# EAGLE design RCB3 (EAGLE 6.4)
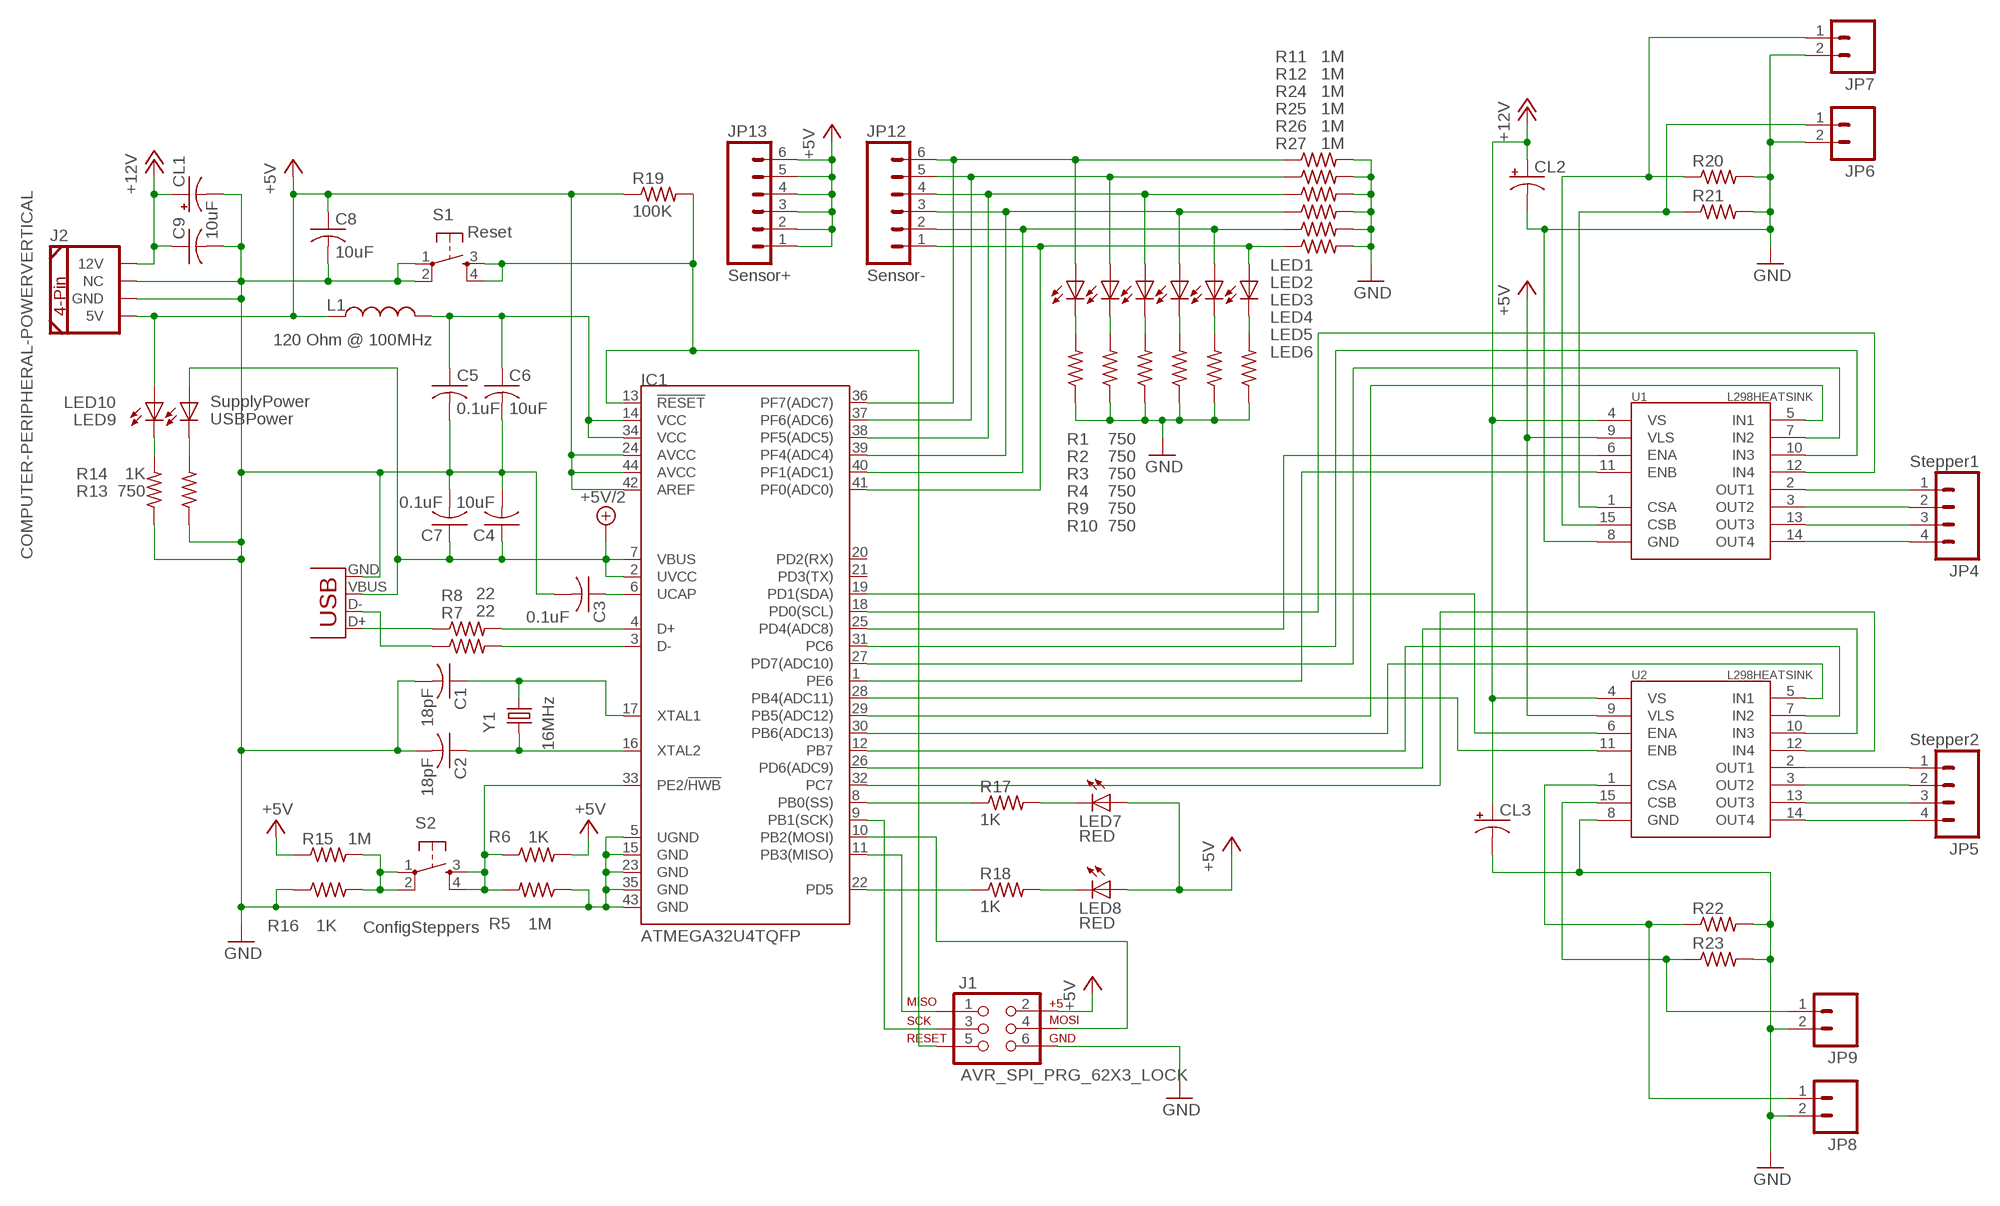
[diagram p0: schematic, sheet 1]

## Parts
C1  18pF  C-USC0603  [C0603]
C2  18pF  C-USC0603  [C0603]
C3  0.1uF  C-USC0603  [C0603]
C4  10uF  C-USC0805  [C0805]
C5  0.1uF  C-USC0603  [C0603]
C6  10uF  C-USC0805  [C0805]
C7  0.1uF  C-USC0603  [C0603]
C8  10uF  C-USC0805  [C0805]
C9  10uF  C-USC0805  [C0805]
CL1  CAP_G  [PANASONIC_G]
CL2  CAP_G  [PANASONIC_G]
CL3  CAP_G  [PANASONIC_G]
IC1  ATMEGA32U4TQFP  [SPARKFUN-DIGITALIC_TQFP44]
J1  AVR_SPI_PRG_62X3_LOCK  [2X3_LOCK]
J2  COMPUTER-PERIPHERAL-POWERVERTICAL  [COMPUTER-PERIPHERAL-POWER]
JP1  USBPTH-VERTICAL  [USB-B-PTH-VERTICAL]
JP4  Stepper1  M04POLAR  [MOLEX-1X4]
JP5  Stepper2  M04POLAR  [MOLEX-1X4]
JP6  M02LOCK  [1X02_LOCK]
JP7  M02LOCK  [1X02_LOCK]
JP8  M02LOCK  [1X02_LOCK]
JP9  M02LOCK  [1X02_LOCK]
JP12  Sensor-  M06LOCK  [1X06_LOCK]
JP13  Sensor+  M06LOCK  [1X06_LOCK]
L1  120 Ohm @ 100MHz  INDUCTOR0603  [0603]
LED1  GREEN  LED-GREEN0603  [LED-0603]
LED2  GREEN  LED-GREEN0603  [LED-0603]
LED3  GREEN  LED-GREEN0603  [LED-0603]
LED4  GREEN  LED-GREEN0603  [LED-0603]
LED5  GREEN  LED-GREEN0603  [LED-0603]
LED6  GREEN  LED-GREEN0603  [LED-0603]
LED7  RED  LED0603  [LED-0603]
LED8  RED  LED0603  [LED-0603]
LED9  USBPower  LED0603  [LED-0603]
LED10  SupplyPower  LED0603  [LED-0603]
R1  750  R-US_R0603  [R0603]
R2  750  R-US_R0603  [R0603]
R3  750  R-US_R0603  [R0603]
R4  750  R-US_R0603  [R0603]
R5  1M  R-US_R0603  [R0603]
R6  1K  R-US_R0603  [R0603]
R7  22  R-US_R0603  [R0603]
R8  22  R-US_R0603  [R0603]
R9  750  R-US_R0603  [R0603]
R10  750  R-US_R0603  [R0603]
R11  1M  R-US_R0603  [R0603]
R12  1M  R-US_R0603  [R0603]
R13  750  R-US_R0603  [R0603]
R14  1K  R-US_R0603  [R0603]
R15  1M  R-US_R0603  [R0603]
R16  1K  R-US_R0603  [R0603]
R17  1K  R-US_R0603  [R0603]
R18  1K  R-US_R0603  [R0603]
R19  100K  R-US_R0603  [R0603]
R20  R-US_R0603  [R0603]
R21  R-US_R0603  [R0603]
R22  R-US_R0603  [R0603]
R23  R-US_R0603  [R0603]
R24  1M  R-US_R0603  [R0603]
R25  1M  R-US_R0603  [R0603]
R26  1M  R-US_R0603  [R0603]
R27  1M  R-US_R0603  [R0603]
S1  Reset  TAC_SWITCHSMD  [TACTILE_SWITCH_SMD]
S2  ConfigSteppers  TAC_SWITCHSMD  [TACTILE_SWITCH_SMD]
U1  L298HEATSINK  [MULTIWATT15_6400BGHEATSINK]
U2  L298HEATSINK  [MULTIWATT15_6400BGHEATSINK]
Y1  16MHz  CRYSTALHC49UV  [HC49U-V]

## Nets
+5V: C8.1 IC1.24(AVCC) IC1.42(AREF) IC1.44(AVCC) J1.2 J2.5V JP13.1 JP13.2 JP13.3 JP13.4 JP13.5 JP13.6 L1.1 LED7.A LED8.A LED10.A R6.2 R15.1 R19.1 U1.9(VLS) U2.9(VLS)
+5V/2: C4.1 C7.1 IC1.2(UVCC) IC1.7(VBUS) JP1.VBUS LED9.A
+12V: C9.1 CL1.+(CAP+) CL2.+(CAP+) CL3.+(CAP+) J2.12V U1.4(VS) U2.4(VS)
GND: C1.2 C2.2 C3.2 C4.2 C5.2 C6.2 C7.2 C8.2 C9.2 CL1.-(CAP-) CL2.-(CAP-) CL3.-(CAP-) IC1.5(UGND) IC1.15(GND) IC1.23(GND) IC1.35(GND) IC1.43(GND) J1.6 J2.GND J2.NC JP1.GND JP6.2 JP7.2 JP8.2 JP9.2 R1.1 R2.1 R3.1 R4.1 R5.1 R9.1 R10.1 R11.2 R12.2 R13.1 R14.1 R16.1 R20.2 R21.2 R22.2 R23.2 R24.2 R25.2 R26.2 R27.2 S1.1 S1.2 U1.8(GND) U2.8(GND)
N$1: IC1.11(PB3(MISO)) J1.1
N$2: IC1.9(PB1(SCK)) J1.3
N$3: IC1.10(PB2(MOSI)) J1.4
N$4: IC1.13(!RESET) J1.5 R19.2 S1.3 S1.4
N$5: IC1.41(PF0(ADC0)) JP12.1 LED6.A R27.1
N$6: IC1.40(PF1(ADC1)) JP12.2 LED5.A R26.1
N$7: IC1.39(PF4(ADC4)) JP12.3 LED4.A R25.1
N$8: IC1.38(PF5(ADC5)) JP12.4 LED3.A R24.1
N$9: JP1.D+ R8.1
N$10: IC1.4(D+) R8.2
N$11: IC1.3(D-) R7.2
N$12: JP1.D- R7.1
N$13: C2.1 IC1.16(XTAL2) Y1.1
N$14: C1.1 IC1.17(XTAL1) Y1.2
N$15: IC1.33(PE2/!HWB) R5.2 R6.1 S2.3 S2.4
N$16: C3.1 IC1.6(UCAP)
N$17: R15.2 R16.2 S2.1 S2.2
N$18: LED8.C R18.2
N$19: LED7.C R17.2
N$20: LED1.C R1.2
N$21: LED2.C R2.2
N$22: C5.1 C6.1 IC1.14(VCC) IC1.34(VCC) L1.2
N$23: LED9.C R13.2
N$24: LED10.C R14.2
N$25: JP5.1 U2.2(OUT1)
N$26: JP5.3 U2.13(OUT3)
N$27: JP5.2 U2.3(OUT2)
N$28: JP5.4 U2.14(OUT4)
N$29: JP4.4 U1.14(OUT4)
N$30: JP4.3 U1.13(OUT3)
N$31: JP4.2 U1.3(OUT2)
N$32: JP4.1 U1.2(OUT1)
N$33: IC1.22(PD5) R18.1
N$34: IC1.8(PB0(SS)) R17.1
N$37: JP8.1 R22.1 U2.1(CSA)
N$38: JP9.1 R23.1 U2.15(CSB)
N$39: JP6.1 R21.1 U1.1(CSA)
N$40: JP7.1 R20.1 U1.15(CSB)
N$41: IC1.29(PB5(ADC12)) U1.5(IN1)
N$42: IC1.27(PD7(ADC10)) U1.7(IN2)
N$43: IC1.31(PC6) U1.10(IN3)
N$44: IC1.18(PD0(SCL)) U1.12(IN4)
N$45: IC1.30(PB6(ADC13)) U2.5(IN1)
N$46: IC1.12(PB7) U2.7(IN2)
N$47: IC1.26(PD6(ADC9)) U2.10(IN3)
N$48: IC1.32(PC7) U2.12(IN4)
N$49: IC1.36(PF7(ADC7)) JP12.6 LED1.A R11.1
N$50: IC1.37(PF6(ADC6)) JP12.5 LED2.A R12.1
N$51: IC1.25(PD4(ADC8)) U1.6(ENA)
N$52: IC1.1(PE6) U1.11(ENB)
N$53: IC1.19(PD1(SDA)) U2.6(ENA)
N$54: IC1.28(PB4(ADC11)) U2.11(ENB)
N$55: LED3.C R3.2
N$56: LED4.C R4.2
N$57: LED5.C R9.2
N$58: LED6.C R10.2
Unconnected: IC1.20(PD2(RX)) IC1.21(PD3(TX))

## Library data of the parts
C1-C4 C6 C8 = resistor:C-US: CAPACITOR, American symbol
C5 C7 C9 = rcl:C-US: CAPACITOR, American symbol
CL1-CL3 = PanasonicSMDCapLib:CAP_G: Panasonic Aluminum Electrolytic Capacitors/ HA
IC1 = SparkFun-DigitalIC:ATMEGA32U4: Atmel 44-pin 8-bit Microcontroller with 32KBytes of ISP Flash and USB Controller
J1 = SparkFun-Connectors:AVR_SPI_PRG_6: AVR ISP 6 Pin This is the reduced ISP connector for AVR programming. Common on Arduino. This footprint will take up less PCB space and can be used with a 10-pin to 6-pin adapter such as SKU: BOB-08508
J2 = SparkFun-Connectors:COMPUTER-PERIPHERAL-POWER
JP1 = SparkFun-Connectors:USB: USB Connectors USB-B-PTH is fully proven SKU : PRT-00139/CONN-08278 USB-miniB is fully proven SKU : PRT-00587 USB-A-PCB is untested. USB-A-H is throughly reviewed, but untested. Spark Fun Electronics SKU : PRT-00437 USB-B-SMT is throughly reviewed, but untested. Needs silkscreen touching up.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
JP4 JP5 = SparkFun-Connectors:M04: Header 4 Standard 4-pin 0.1" header. Use with straight break away headers (SKU : PRT-00116), right angle break away headers (PRT-00553), swiss pins (PRT-00743), machine pins (PRT-00117), and female headers (PRT-00115). Molex polarized connector foot print use with SKU : PRT-08231 with associated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
JP6-JP9 = SparkFun-Connectors:M02: Header 2
JP12 JP13 = SparkFun-Connectors:M06: Header 6 Standard 6-pin 0.1" header. Use with straight break away headers (SKU : PRT-00116), right angle break away headers (PRT-00553), swiss pins (PRT-00743), machine pins (PRT-00117), and female headers (PRT-00115). Molex polarized connector foot print use with SKU : PRT-08094 with associated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
L1 = SparkFun-Passives:INDUCTOR: Inductors
LED1-LED6 = SparkFun-LED:LED-GREEN: Various green LEDs; PROD_ID: DIO-00821
LED7-LED10 = SparkFun:LED: LEDs
R1-R6 R9-R12 R24-R27 = resistor:R-US_: RESISTOR, American symbol
R7 R8 R13-R23 = rcl:R-US_: RESISTOR, American symbol
S1 S2 = SparkFun:TAC_SWITCH: Momentary Switch Button commonly used for reset or general input. Spark Fun Electronics SKU : COM-00097
U1 U2 = SparkFun-PowerIC:L298: L298 Dual Full Bridge Driver
Y1 = SparkFun:CRYSTAL: Crystals

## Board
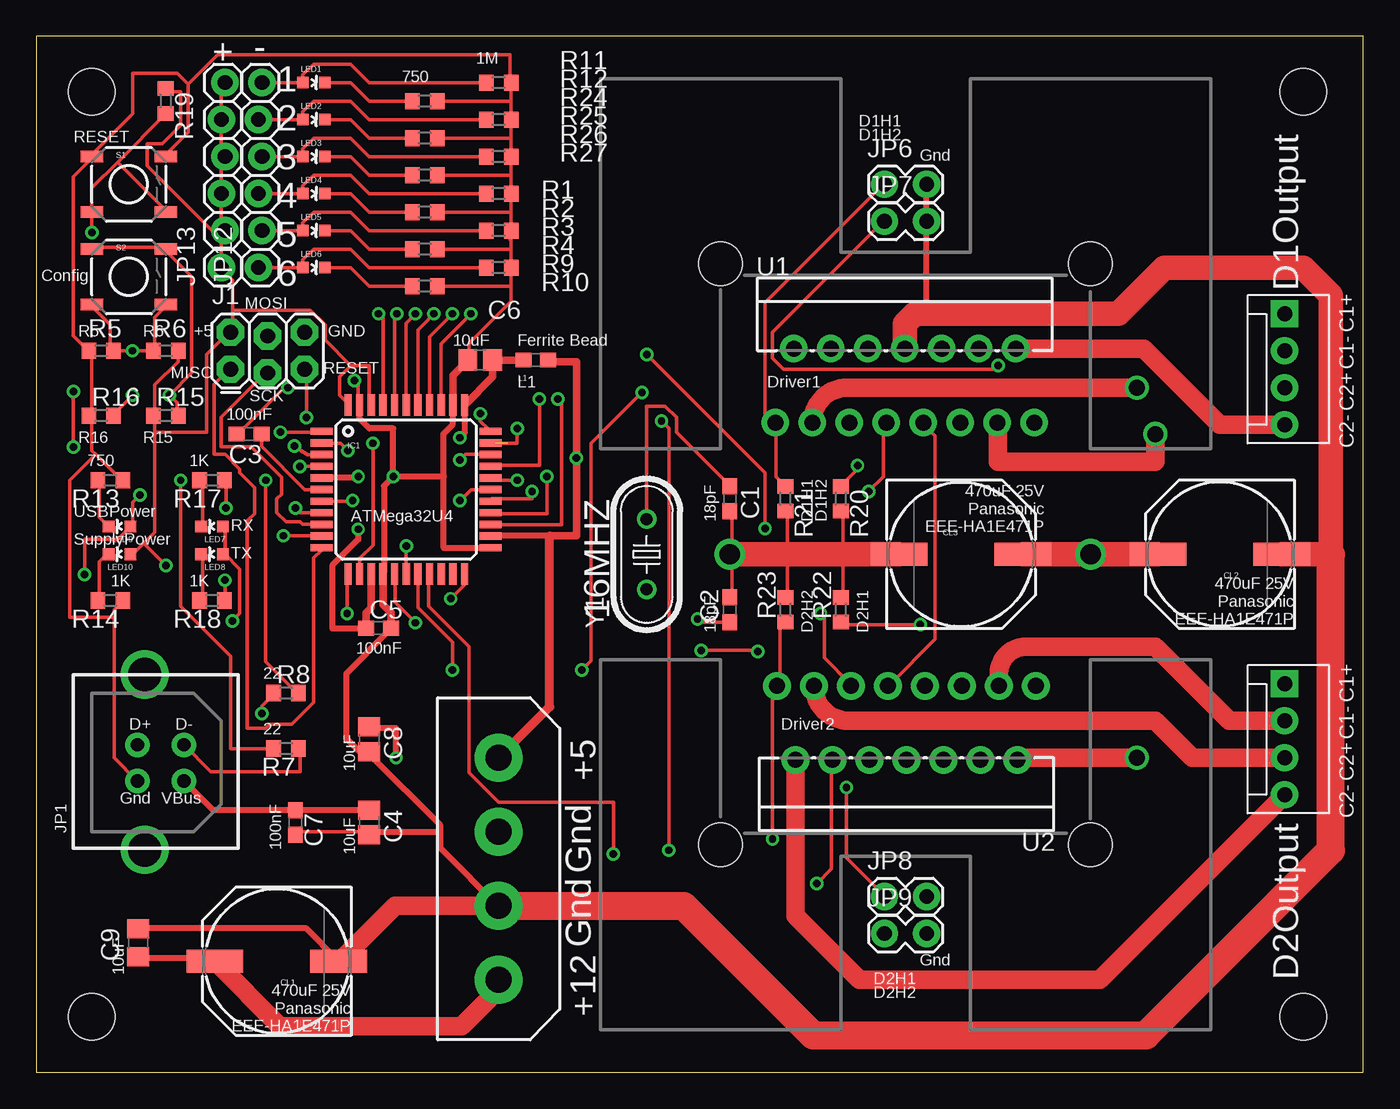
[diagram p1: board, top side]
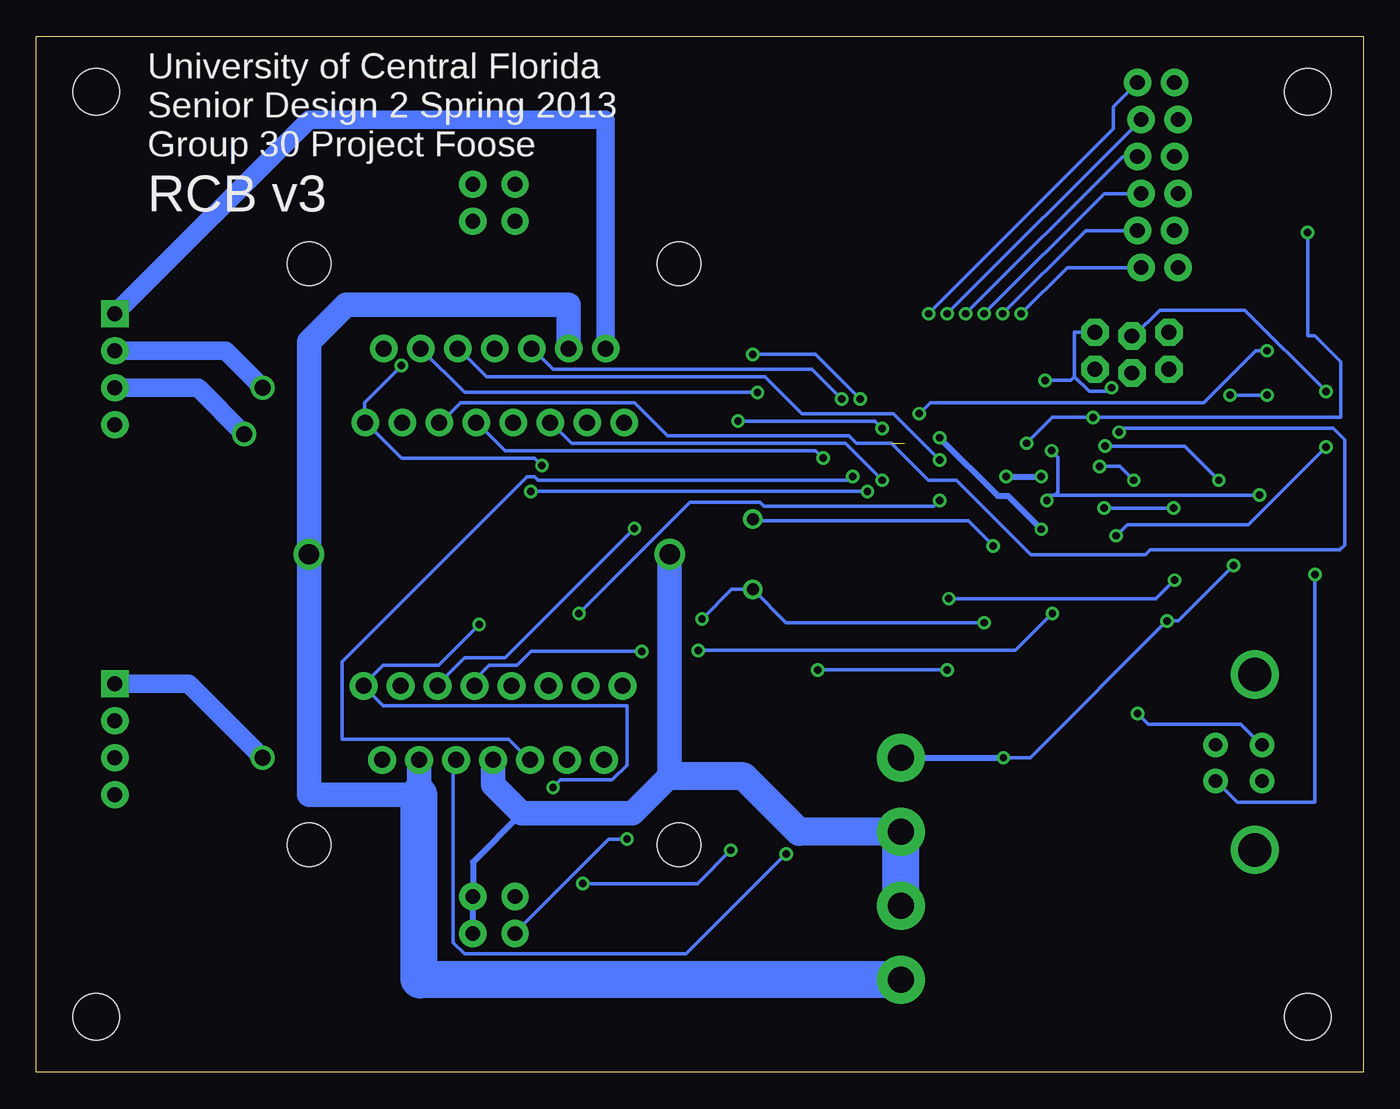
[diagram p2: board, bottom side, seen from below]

Size 91.11 x 71.11 mm. Coordinates in mm from the lower left corner, seen from the top.
Outline: 0,0 91.11,0 91.11,71.11 0,71.11 0,0
Copper layers (1*16): Top 0.035mm / dielectric 1.5mm / Bottom 0.035mm
Design rules "default *": minimum track width 10mil, minimum drill 20mil, track to track 8mil, track to pad 10mil, pad to pad 10mil, via to via 10mil, smd to smd 8mil, copper to edge 40mil, drill to drill 8mil, minimum pad ring 10mil, minimum via ring 8mil, stop-mask expansion 4mil, vias tented up to drill 0mil, thermal gap 10mil
Holes 3.2 mm at 3.81,3.81 3.81,67.31 87,67.31 87,3.81

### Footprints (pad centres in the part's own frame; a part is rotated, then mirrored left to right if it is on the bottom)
C0603 = smd 1.1 x 1: 1 -0.85,0; 2 0.85,0
C0805 = smd 1.3 x 1.5: 1 -0.85,0; 2 0.85,0
C0805' = smd 1.3 x 1.5: 1 -0.95,0; 2 0.95,0
PANASONIC_G = smd 3.9 x 1.6: + 4.25,0; - -4.25,0
SPARKFUN-DIGITALIC_TQFP44 = smd 1.5 x 0.5: 1 -5.8,4; 2 -5.8,3.2; 3 -5.8,2.4; 4 -5.8,1.6; 5 -5.8,0.8; 6 -5.8,0; 7 -5.8,-0.8; 8 -5.8,-1.6; 9 -5.8,-2.4; 10 -5.8,-3.2; 11 -5.8,-4; 23 5.8,-4; 24 5.8,-3.2; 25 5.8,-2.4; 26 5.8,-1.6; 27 5.8,-0.8; 28 5.8,0; 29 5.8,0.8; 30 5.8,1.6; 31 5.8,2.4; 32 5.8,3.2; 33 5.8,4 | smd 0.5 x 1.5: 12 -4,-5.8; 13 -3.2,-5.8; 14 -2.4,-5.8; 15 -1.6,-5.8; 16 -0.8,-5.8; 17 0,-5.8; 18 0.8,-5.8; 19 1.6,-5.8; 20 2.4,-5.8; 21 3.2,-5.8; 22 4,-5.8; 34 4,5.8; 35 3.2,5.8; 36 2.4,5.8; 37 1.6,5.8; 38 0.8,5.8; 39 0,5.8; 40 -0.8,5.8; 41 -1.6,5.8; 42 -2.4,5.8; 43 -3.2,5.8; 44 -4,5.8
2X3_LOCK = drill 1.016 pad 1.88 octagon: 1 0,0; 2 0,2.54; 3 2.54,-0.254; 4 2.54,2.286; 5 5.08,0; 6 5.08,2.54
COMPUTER-PERIPHERAL-POWER = drill 1.778 pad 3.302: 5V 7.62,0; 12V -7.62,0; GND 2.54,0; NC -2.54,0
USB-B-PTH-VERTICAL = drill 0.914 pad 1.676: D+ 4.826,4.394; D- 4.826,7.595; GND 7.315,4.394; VBUS 7.315,7.595 | drill 2.286: P$1 0,4.902; P$2 12.04,4.902
MOLEX-1X4 = drill 1.016 pad 1.88 square: 1 0,0 | drill 1.016 pad 1.88: 2 2.54,0; 3 5.08,0; 4 7.62,0
1X02_LOCK = drill 1.016 pad 1.88: 1 -0.178,0; 2 2.718,0
1X06_LOCK = drill 1.016 pad 1.88: 1 0,0; 2 2.54,-0.254; 3 5.08,0; 4 7.62,-0.254; 5 10.16,0; 6 12.7,-0.254
0603 = smd 1.1 x 1: 1 -0.85,0; 2 0.85,0
LED-0603 = smd 0.8 x 0.8: A 0,-0.75; C 0,0.75
R0603 = smd 1 x 1.1: 1 -0.85,0; 2 0.85,0
TACTILE_SWITCH_SMD = smd 1.524 x 0.762: 1 -2.54,1.905; 2 2.54,1.905; 3 -2.54,-1.905; 4 2.54,-1.905
MULTIWATT15_6400BGHEATSINK = drill 1.1 pad 1.9: 1 -8.95,-2.39; 2 -7.68,2.69; 3 -6.41,-2.39; 4 -5.14,2.69; 5 -3.87,-2.39; 6 -2.6,2.69; 7 -1.33,-2.39; 8 -0.06,2.69; 9 1.21,-2.39; 10 2.48,2.69; 11 3.75,-2.39; 12 5.02,2.69; 13 6.29,-2.39; 14 7.56,2.69; 15 8.83,-2.39 | hole 2.997: -12.7,8.509; 12.7,8.509
HC49U-V = drill 0.813: 1 -2.413,0; 2 2.413,0

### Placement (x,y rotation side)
C1  47.62,39.37 270 top
C2  47.62,31.75 90 top
C3  14.61,43.81 180 top
C4  22.86,17.14 270 top
C5  23.5,30.48 0 top
C6  30.48,48.9 180 top
C7  17.78,17.14 270 top
C8  22.86,22.86 270 top
C9  10uF  [C0805']  6.99,8.89 90 top
CL1  16.51,7.62 180 top
CL2  81.28,35.56 180 top
CL3  63.5,35.56 0 top
IC1  25.4,40.01 0 top
J1  13.34,48.26 0 top
J2  31.75,13.97 90 top
JP1  2.54,27.3 270 top
JP4  85.72,52.07 270 top
JP5  85.72,26.67 270 top
JP6  58.42,60.96 0 top
JP7  58.42,58.42 0 top
JP8  58.42,12.06 0 top
JP9  58.42,9.53 0 top
JP12  15.24,55.24 90 top
JP13  12.7,55.24 90 top
L1  34.29,48.9 180 top
LED1  19.05,67.94 270 top
LED2  19.05,65.41 270 top
LED3  19.05,62.87 270 top
LED4  19.05,60.33 270 top
LED5  19.05,57.78 270 top
LED6  19.05,55.24 270 top
LED7  12.06,37.47 90 top
LED8  12.06,35.56 90 top
LED9  5.71,37.47 90 top
LED10  5.71,35.56 90 top
R1  26.67,66.67 180 top
R2  26.67,64.14 180 top
R3  26.67,61.59 180 top
R4  26.67,59.05 180 top
R5  4.45,49.53 0 top
R6  8.89,49.53 0 top
R7  17.14,22.23 180 top
R8  17.14,26.04 0 top
R9  26.67,56.52 180 top
R10  26.67,53.98 180 top
R11  31.75,67.94 0 top
R12  31.75,65.41 0 top
R13  5.08,40.64 180 top
R14  5.08,32.38 180 top
R15  8.89,45.09 0 top
R16  4.45,45.09 0 top
R17  12.06,40.64 180 top
R18  12.06,32.38 180 top
R19  8.89,66.67 270 top
R20  55.24,39.37 270 top
R21  51.44,39.37 270 top
R22  55.24,31.75 90 top
R23  51.44,31.75 90 top
R24  31.75,62.87 0 top
R25  31.75,60.33 0 top
R26  31.75,57.78 0 top
R27  31.75,55.24 0 top
S1  6.35,60.96 0 top
S2  6.35,54.61 0 top
U1  59.69,46.99 0 top
U2  59.69,24.13 180 top
Y1  41.91,35.56 90 top

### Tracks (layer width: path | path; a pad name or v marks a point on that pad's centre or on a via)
+5V  (via drill 0.51)
  Top 0.254: 12.7,57.15 JP13.1 12.7,55.12 13.46,54.36 13.46,52.32 | 12.7,57.15 12.7,57.53 JP13.2 | JP13.2 12.7,58.04 JP13.3 12.7,62.61 JP13.4 12.7,63.12 JP13.5 12.7,67.69 JP13.6 | 7.37,36.32 8.13,37.08 8.13,43.94 | 7.37,36.32 6.6,35.56 LED10.A | 8.13,43.94 8.13,44.96 R15.1 8.13,45.21 8.13,47.18 9.74,48.79 R6.2 9.65,49.53 | 12.7,57.15 7.62,62.23 7.62,63.75 8.64,63.75 9.91,65.02 9.91,67.31 8.89,67.31 R19.1 | 12.7,57.15 JP13.2 | 21.59,48.51 20.83,47.75 20.83,46.48 21.34,45.97 IC1.44 | 21.59,48.51 22.86,48.51 22.86,45.97 IC1.42 | 21.59,48.51 19.81,50.29 19.81,51.31 18.8,52.32 13.46,52.32 | 13.46,52.32 13.46,50.8 J1.2 13.21,50.8 11.68,49.28 11.68,43.94 8.13,43.94 | U2.9 58.67,26.67 61.72,29.72 61.72,43.69 60.96,44.45 U1.9 | 35.31,48.77 L1.1 | 31.24,36.83 IC1.24 | 12.95,35.56 12.95,37.34 LED7.A | 12.95,35.56 13.97,34.54 13.97,31.5 v13.46,30.99 | 12.95,35.56 LED8.A | 22.86,23.62 C8.1 | v8.89,34.8 7.37,36.32
  Top 0.406: 22.86,23.62 24.7,23.62 v24.7,21.59 | 35.24,36.83 31.2,36.83 IC1.24
  Top 0.508: 35.24,36.83 37.08,36.83 v37.08,42.16 37.08,48.77 35.31,48.77
  Top 0.61: J2.5V 35.24,25.08 35.24,36.83
  Bottom 0.254: v24.7,21.59 22.86,21.59 v13.46,30.99 12.7,30.99 v8.89,34.8 | v37.08,42.16 37.59,42.67 58.93,42.67 60.71,44.45 U1.9
  Bottom 0.406: J2.5V v24.7,21.59
+5V/2  (via drill 0.51)
  Top 0.254: v21.4,42.67 20.89,43.18 19.81,43.18 IC1.2 | v3.3,34.16 3.3,36.58 5.59,36.58 6.35,37.34 LED9.A 6.6,37.59 6.6,39.12 v7.11,39.62 | IC1.7 21.68,39.2 arc90 v21.72,39.24
  Top 0.406: C4.1 C7.1 12.13,18 JP1.VBUS
  Bottom 0.254: v3.3,34.16 3.3,18.54 8.64,18.54 9.91,19.81 JP1.VBUS | v7.11,39.62 21.27,39.62 | 21.27,39.62 21.34,39.62 arc-90 v21.72,39.24 | v21.4,42.67 20.95,42.23 20.95,39.94 arc90 21.27,39.62
+12V  (via drill 1.4)
  Top 0.254: 12.19,7.87 12.19,7.62 CL1.+ | 7.11,7.87 C9.1
  Top 0.406: 7.11,7.87 12.01,7.87 CL1.+
  Top 1.27: CL1.+ 16.7,3.17 29.21,3.17 31.75,5.71 J2.12V
  Top 1.676: CL2.+ CL3.+ v72.39,35.56
  Bottom 1.27: 64.77,6.35 64.83,6.41
  Bottom 1.676: U1.4 54.55,52.7 69.85,52.7 72.39,50.16 v72.39,35.56 72.39,19.05 64.83,19.05 U2.4
  Bottom 2.54: J2.12V 64.77,6.35 | 64.83,6.41 64.83,19.05
GND  (via drill 0.51, 1.4)
  Top 0.254: R27.2 32.6,56.52 | 32.6,56.52 32.6,57.15 | 32.6,57.15 R26.2 32.6,59.05 | 32.6,59.05 R25.2 32.6,61.59 | 32.6,61.59 R24.2 32.6,64.14 | 32.6,64.14 R12.2 32.6,66.67 | 32.6,66.67 R11.2 32.51,68.07 32.51,69.85 12.45,69.85 10.41,67.82 | R9.1 32.6,56.52 | R4.1 32.6,59.05 | R3.1 32.6,61.59 | R2.1 32.6,64.14 | R1.1 32.6,66.67 | R10.1 32.6,53.98 R27.2 | 5.33,31.24 5.33,21.59 JP1.GND | 5.33,31.24 5.33,31.75 5.84,32.26 R14.1 | 6.86,9.91 C9.2 | 4.06,42.42 3.81,42.67 3.81,44.96 R16.1 3.81,45.21 3.81,49.53 R5.1 3.56,49.53 2.54,50.55 2.54,61.47 3.81,62.74 S1.1 3.81,62.99 6.6,65.79 6.6,68.58 9.65,68.58 10.41,67.82 | 4.06,42.42 5.84,40.64 R13.1 | 10.41,67.82 10.41,64.52 8.89,62.99 S1.2 | 5.33,31.24 2.29,31.24 2.29,40.64 4.06,42.42 | C2.2 47.75,32.77 47.75,34.8 v47.62,35.56 47.75,36.32 47.75,38.35 C1.2 47.75,38.61 | R23.2 51.56,32.77 51.56,35.56 51.56,38.35 R21.2 | R22.2 55.37,32.77 55.37,35.56 55.37,38.35 R20.2 | 32.51,57.15 32.6,57.15 | C7.2 17.78,16.51 22.86,16.51 C4.2 | 20.83,7.62 CL1.- | v17.27,46.99 17.02,46.99 13.97,43.94 C3.2 | 23.88,34.29 IC1.15 | v21.84,47.5 22.1,47.24 22.1,45.97 IC1.43 | 24.13,30.23 24.13,30.48 C5.2 | C6.2 29.72,49.02 29.72,50.04 32.6,52.92 R27.2 | 31.88,11.24 J2.NC | 22.61,21.59 22.86,21.84 C8.2 22.61,21.59
  Top 0.406: 60.33,52.07 61.14,52.88 JP7.2 JP6.2 | v24.51,40.89 24.51,44.2 22.86,44.2 22.2,44.86 IC1.43 | 23.88,34.29 23.88,40.26 v24.51,40.89 | 22.61,21.59 21.27,22.92 21.27,27.37 24.13,30.23 | 22.86,21.84 27.75,16.95 27.75,16.51 | 27.75,16.51 27.75,15.37 31.88,11.24 | v22.1,40.89 22.01,40.8 IC1.5 | IC1.23 27.96,36.01 27.96,40.89 27.94,40.89 | 22.86,16.51 27.75,16.51 | 27.94,40.89 v24.51,40.89 | IC1.35 28.57,45.78 28.57,44.45 27.94,43.81 27.94,40.89 | 6.86,9.91 18.47,9.91 CL1.-
  Top 0.508: C6.2 28.6,47.87 IC1.35 | IC1.15 23.8,32.08 24.34,31.54 C5.2
  Top 1.27: 20.83,7.62 24.64,11.43 J2.NC
  Top 1.676: CL2.- 88.9,35.56 88.9,53.34 87,55.24 77.47,55.24 74.3,52.07 60.33,52.07 59.63,51.38 U1.8 | CL3.- 55.37,35.56 51.56,35.56 v47.62,35.56
  Top 1.93: J2.NC 44.45,11.43 53.34,2.54 76.2,2.54 88.9,15.24 88.9,35.56
  Bottom 0.254: v17.27,46.99 17.53,46.74 18.8,46.74 19.81,47.75 | 19.81,47.75 19.81,50.8 J1.6 | 19.81,47.75 20.07,47.5 v21.84,47.5
  Bottom 0.406: 57.78,17.78 61.14,14.43 JP8.2 JP9.2 | v24.51,40.89 v22.1,40.89
  Bottom 1.676: v47.62,35.56 47.62,20.32 50.16,17.78 57.78,17.78 59.75,19.75 U2.8
  Bottom 1.93: J2.GND 38.73,16.51 42.55,20.32 47.62,20.32
  Bottom 2.54: J2.NC J2.GND
N$1
  Top 0.254: IC1.11 19.56,35.81 19.05,35.31 19.05,25.4 17.53,23.88 16,23.88 15.75,23.62 14.48,23.62 14.48,37.85 14.99,38.35 14.99,40.13 13.97,41.15 13.97,41.4 12.95,42.42 12.19,42.42 12.19,47.24 13.21,48.26 J1.1
N$2
  Top 0.254: 19.56,37.59 IC1.9 18.27,37.6 18.1,37.78 17.14,37.78 16.51,38.42 16.51,39.37 16.83,39.69 16.83,40.83 14.73,42.93 12.7,42.93 12.7,44.96 15.75,48.01 J1.3
N$3  (via drill 0.51)
  Top 0.254: v16.95,36.83 19.81,36.83 IC1.10 | v2.54,46.74 v2.54,42.93
  Bottom 0.254: v16.95,36.83 16.19,37.59 7.87,37.59 v2.54,42.93 | v2.54,46.74 8.13,52.32 13.97,52.32 15.75,50.55 J1.4
N$4  (via drill 0.51)
  Top 0.254: 5.59,62.48 3.81,60.71 S1.3 v3.81,57.66 | 5.59,62.48 8.89,65.79 R19.2 | 5.59,62.48 8.89,59.18 S1.4 | v23.11,43.18 23.11,36.2 22.2,35.28 IC1.13 | v18.54,44.96 18.54,48.26 J1.5
  Bottom 0.254: v23.11,43.18 21.34,44.96 v18.54,44.96 1.52,44.96 1.52,48.77 3.3,50.55 3.81,50.55 v3.81,57.66
N$5  (via drill 0.51)
  Top 0.254: JP12.1 LED6.A 18.3,55.77 19.05,56.52 21.59,56.52 22.86,55.24 R27.1 | IC1.41 23.8,51.77 v23.5,52.07
  Bottom 0.254: v23.5,52.07 20.32,55.24 JP12.1
N$6  (via drill 0.51)
  Top 0.254: JP12.2 LED5.A 18.3,58.3 19.05,59.05 21.59,59.05 22.86,57.78 R26.1 | IC1.40 24.6,51.91 v24.77,52.07
  Bottom 0.254: v24.77,52.07 19.05,57.78 JP12.2
N$7  (via drill 0.51)
  Top 0.254: JP12.3 LED4.A 18.3,60.84 19.05,61.59 21.59,61.59 22.86,60.33 R25.1 | IC1.39 25.4,51.44 v26.04,52.07
  Bottom 0.254: v26.04,52.07 17.78,60.33 JP12.3
N$8  (via drill 0.51)
  Top 0.254: JP12.4 LED3.A 18.3,63.38 19.05,64.14 21.59,64.14 22.86,62.87 R24.1 | IC1.38 26.2,50.97 v27.3,52.07
  Bottom 0.254: v27.3,52.07 16.51,62.87 JP12.4
N$9  (via drill 0.51)
  Top 0.254: v15.49,24.64 15.49,25.15 16.26,25.91 R8.1
  Bottom 0.254: v15.49,24.64 14.73,23.88 8.38,23.88 7.11,22.61 JP1.D+
N$10  (via drill 0.51)
  Top 0.254: v15.75,40.64 15.75,28.19 17.78,26.16 R8.2 | IC1.4 18.11,41.6 v18.1,41.59
  Bottom 0.254: v18.1,41.59 16.7,41.59 v15.75,40.64
N$11  (via drill 0.51)
  Top 0.254: v9.91,40.64 9.91,32 13.34,28.57 13.34,22.23 R7.2 | 19.56,42.42 IC1.3 18.62,42.41 v17.72,42.99
  Bottom 0.254: v9.91,40.64 12.26,42.99 v17.72,42.99
N$12
  Top 0.254: R7.1 18.1,22.12 18.1,20.64 11.98,20.64 JP1.D-
N$13  (via drill 0.51)
  Top 0.254: v26.04,30.86 24.64,32.26 24.64,34.04 IC1.16 | C2.1 45.62,30.9 v45.4,31.11
  Bottom 0.254: v45.4,31.11 43.37,33.15 Y1.1 39.62,30.86 v26.04,30.86
N$14  (via drill 0.51)
  Top 0.254: Y1.2 41.91,45.72 43.18,45.72 43.94,44.96 43.94,43.94 47.5,40.39 C1.1 | v25.4,36.13 IC1.17
  Bottom 0.254: v25.4,36.13 27.11,37.85 41.91,37.85 Y1.2
N$15  (via drill 0.51)
  Top 0.254: v30.48,45.21 30.48,44.7 30.99,44.2 IC1.33 | S2.3 3.81,52.58 5.08,51.31 5.08,49.53 R5.2 v6.6,49.53 R6.1 8.13,49.53 8.13,51.82 8.89,52.58 S2.4
  Bottom 0.254: v30.48,45.21 29.72,45.97 10.92,45.97 7.37,49.53 v6.6,49.53
N$16
  Top 0.254: 15.49,43.69 C3.1 15.46,42.97 18.41,40.01 IC1.6
N$17  (via drill 0.51)
  Top 0.254: v6.6,46.48 5.33,45.21 R16.2 | R15.2 9.65,45.21 9.65,45.97 v9.14,46.48 10.67,48.01 10.67,54.61 8.89,56.39 S2.2 8.89,56.64 3.81,56.64 S2.1
  Bottom 0.254: v9.14,46.48 v6.6,46.48
N$18
  Top 0.254: LED8.C 11.43,35.56 11.43,32.51 R18.2
N$19
  Top 0.254: LED7.C 11.43,37.59 11.43,40.64 R17.2
N$20
  Top 0.254: LED1.C 21.59,67.94 22.86,66.67 R1.2
N$21
  Top 0.254: LED2.C 21.59,65.41 22.86,64.14 R2.2
N$22  (via drill 0.51)
  Top 0.254: IC1.14 22.86,34.2 22.86,31.75
  Top 0.406: C5.1 20.32,30.48 20.32,34.8 22.1,36.58 v22.1,37.27 | IC1.34 29.4,43.88 v29.08,43.56
  Top 0.508: IC1.34 31.33,47.73 C6.1 L1.2 | IC1.14 23,31.89 22.86,31.75 22.64,31.54 C5.1
  Bottom 0.406: v22.1,37.27 24.38,39.56 25.08,39.56 v29.08,43.56
N$23
  Top 0.254: LED9.C 4.83,37.59 4.32,38.1 4.32,40.64 R13.2
N$24
  Top 0.254: LED10.C 4.83,35.56 4.32,35.05 4.32,32.51 R14.2
N$25  (via drill 1.1)
  Top 1.27: U2.2 67.52,21.59 v75.56,21.59
  Bottom 1.27: JP5.1 80.64,26.67 v75.56,21.59
N$26
  Top 1.27: JP5.3 79.38,21.59 76.83,24.13 55.79,24.13 arc-90 U2.13
N$27
  Top 1.27: JP5.2 81.92,24.13 76.83,29.21 67.94,29.21 arc90 66.1,27.36 U2.3
N$28
  Top 1.27: JP5.4 73.03,6.35 56.52,6.35 52.13,10.73 U2.14
N$29
  Top 1.27: JP4.4 81.28,44.45 76.05,49.68 U1.14
N$30  (via drill 1.1)
  Top 1.27: U1.13 66.04,44.54 66.04,41.91 76.83,41.91 v76.83,43.81
  Bottom 1.27: v76.83,43.81 80.01,46.99 JP4.3
N$31  (via drill 1.1)
  Top 1.27: v75.56,46.99 55.67,46.99 arc90 U1.3
  Bottom 1.27: JP4.2 78.11,49.53 v75.56,46.99
N$32
  Bottom 1.27: JP4.1 72.39,65.41 52.07,65.41 52.01,65.34 U1.2
N$33  (via drill 0.51)
  Top 0.254: v12.95,33.78 12.95,32.51 R18.1 | v28.45,32.51 29.46,33.53 29.46,34.04 IC1.22
  Bottom 0.254: v12.95,33.78 14.22,32.51 v28.45,32.51
N$34  (via drill 0.51)
  Top 0.254: 19.81,38.35 IC1.8 18.11,38.41 v17.78,38.73 | R17.1 13.02,40.64 v13.02,38.73
  Bottom 0.254: v13.02,38.73 v17.78,38.73
N$37  (via drill 0.51)
  Top 0.254: v60.71,30.73 55.37,30.73 R22.1 | v55.63,19.56 55.63,14.73 58.17,12.19 JP8.1
  Bottom 0.254: v60.71,30.73 63.5,27.94 67.31,27.94 68.58,26.67 U2.1 68.58,26.42 67.31,25.15 50.55,25.15 50.55,21.08 51.56,20.07 55.12,20.07 v55.63,19.56
N$38  (via drill 0.51)
  Top 0.254: R23.1 51.31,30.73 51.05,30.48 51.05,26.67 U2.15 50.8,26.42 50.55,26.16 v50.55,16
  Bottom 0.254: v50.55,16 51.82,16 58.17,9.65 JP9.1
N$39
  Top 0.254: R21.1 51.31,40.39 50.8,40.89 50.8,44.45 U1.1 50.55,44.7 50.04,45.21 50.04,52.83 58.17,60.96 JP6.1
N$40  (via drill 0.51)
  Top 0.254: v56.39,41.66 56.39,41.4 55.37,40.39 R20.1 | v66.04,48.51 66.04,48.26 51.31,48.26 50.55,49.02 50.55,50.8 58.17,58.42 JP7.1
  Bottom 0.254: v56.39,41.66 56.9,42.16 66.04,42.16 68.33,44.45 U1.15 68.58,44.7 68.58,45.97 v66.04,48.51
N$41  (via drill 0.51)
  Top 0.254: v33.02,40.64 31.24,40.64 IC1.29
  Bottom 0.254: v33.02,40.64 35.56,43.18 54.36,43.18 55.63,44.45 U1.5
N$42  (via drill 0.51)
  Top 0.254: v34.04,39.88 34.04,39.37 31.24,39.37 IC1.27 | v57.15,39.88 58.17,40.89 58.17,44.45 U1.7
  Bottom 0.254: v57.15,39.88 v34.04,39.88
N$43  (via drill 0.51)
  Top 0.254: IC1.31 30.99,42.42 29.46,42.42 v29.08,42.04
  Bottom 0.254: v29.08,42.04 32.26,45.21 38.54,45.21 41.08,47.75 60.2,47.75 61.98,49.53 U1.10
N$44  (via drill 0.51)
  Top 0.254: IC1.18 26.2,31.9 28.57,29.53 v28.57,27.62 | v41.59,46.67 38.1,43.18 38.1,28.26 v37.47,27.62
  Bottom 0.254: v28.57,27.62 v37.47,27.62 | v41.59,46.67 61.7,46.67 U1.12
N$45  (via drill 0.51)
  Top 0.254: v34.54,46.23 34.54,41.66 31.24,41.66 IC1.30 | v41.91,49.28 50.04,41.15 v50.04,37.34
  Bottom 0.254: v34.54,46.23 37.59,49.28 v41.91,49.28 | v50.04,37.34 58.93,28.45 61.72,28.45 63.5,26.67 U2.5
N$46  (via drill 0.51)
  Top 0.254: v21.34,31.5 21.34,34.04 IC1.12 | v45.66,28.96 49.47,28.96 v49.53,28.89
  Bottom 0.254: v21.34,31.5 23.88,28.96 v45.66,28.96 | v49.53,28.89 57.15,28.89 58.1,27.94 60.01,27.94 61.02,26.93 U2.7
N$47  (via drill 0.51)
  Top 0.254: v35.05,40.89 35.05,38.35 31.24,38.35 IC1.26
  Bottom 0.254: v35.05,40.89 35.31,40.64 56.64,40.64 56.9,40.89 57.4,40.89 70.1,28.19 70.1,22.86 58.67,22.86 57.4,21.59 U2.10
N$48  (via drill 0.51)
  Top 0.254: v33.02,44.2 33.02,43.18 31.24,43.18 IC1.32 | v42.93,44.7 43.43,44.2 v43.43,15.24 | v53.59,12.95 54.61,13.97 54.61,21.34 U2.12
  Bottom 0.254: v33.02,44.2 33.53,44.7 v42.93,44.7 | v43.43,15.24 45.72,12.95 v53.59,12.95
N$49  (via drill 0.51)
  Top 0.254: JP12.6 LED1.A 18.3,68.47 19.05,69.22 21.59,69.22 22.86,67.94 R11.1 | IC1.36 27.8,50.02 v29.84,52.07
  Bottom 0.254: v29.84,52.07 17.14,64.77 17.14,66.29 JP12.6
N$50  (via drill 0.51)
  Top 0.254: JP12.5 LED2.A 18.3,65.92 19.05,66.67 21.59,66.67 22.86,65.41 R12.1 | IC1.37 27,50.49 v28.57,52.07
  Bottom 0.254: v28.57,52.07 JP12.5
N$51  (via drill 0.51)
  Top 0.254: v35.81,46.23 36.07,45.97 36.07,37.59 31.24,37.59 IC1.25
  Bottom 0.254: v35.81,46.23 37.85,48.26 55.63,48.26 56.9,49.53 U1.6
N$52  (via drill 0.51)  (1 unrouted)
  Top 0.254: v16.76,43.94 19.56,43.94 IC1.1
  Bottom 0.254: v16.76,43.94 16.51,44.2 2.03,44.2 1.27,43.43 1.27,36.2 1.59,35.88 14.61,35.88 14.95,35.53 22.83,35.53 27.94,40.64 29.84,40.64 32.38,43.18 34.8,43.18 35.31,43.69 47.75,43.69 50.04,45.97 61.98,45.97 63.25,44.7 U1.11
N$53  (via drill 0.51)
  Top 0.254: v39.62,14.99 39.62,18.54 31.75,18.54 29.72,20.57 29.72,29.21 26.92,32 26.92,34.04 IC1.19
  Bottom 0.254: v39.62,14.99 46.48,8.13 61.72,8.13 62.48,8.89 62.48,21.34 U2.6
N$54  (via drill 0.51)
  Top 0.254: v53.85,31.5 54.1,31.24 54.1,28.45 55.88,26.67 U2.11 | 30.99,39.88 IC1.28 29.84,40.01 v29.08,39.24
  Bottom 0.254: v53.85,31.5 46.23,39.12 41.4,39.12 41.15,38.86 29.46,38.86 v29.08,39.24
N$55
  Top 0.254: LED3.C 21.59,62.87 22.86,61.59 R3.2
N$56
  Top 0.254: R4.2 22.86,59.05 21.59,60.33 LED4.C
N$57
  Top 0.254: R9.2 22.86,56.52 21.59,57.78 LED5.C
N$58
  Top 0.254: LED6.C 21.59,55.24 22.86,53.98 R10.2

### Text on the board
_tsilk: - | + | 1M | 750 | D1H1 | D1H2 | RESET | Gnd | Config | 1 / 2 / 3 / 4 / 5 / 6 | D1Output | MOSI | C1+ | R5 | R6 | +5 | GND | 10uF | Ferrite Bead | MISO | RESET | C1- | L1 | Driver1 | SCK | 100nF | C2+ | R16 | R15 | C2- | 750 | 1K | 470uF 25V / Panasonic / EEE-HA1E471P | USBPower | ATMega32U4 | 18pF | D1H1 | D1H2 | RX | SupplyPower | TX | 470uF 25V / Panasonic / EEE-HA1E471P | 1K | 1K | 16MHZ | 100nF | 18pF | D2H2 | D2H1 | 22 | C1+ | D+ | D- | 22 | Driver2 | C1- | 10uF | +5 | C2+ | Gnd | VBus | C2- | 100nF | 10uF | Gnd | Gnd | 10uF | Gnd | 470uF 25V / Panasonic / EEE-HA1E471P | D2H1 | D2Output | D2H2 | +12
_bsilk: University of Central Florida / Senior Design 2 Spring 2013 / Group 30 Project Foose | RCB v3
